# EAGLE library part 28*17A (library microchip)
CMOS EEPROM 16 K (2 K x 8)
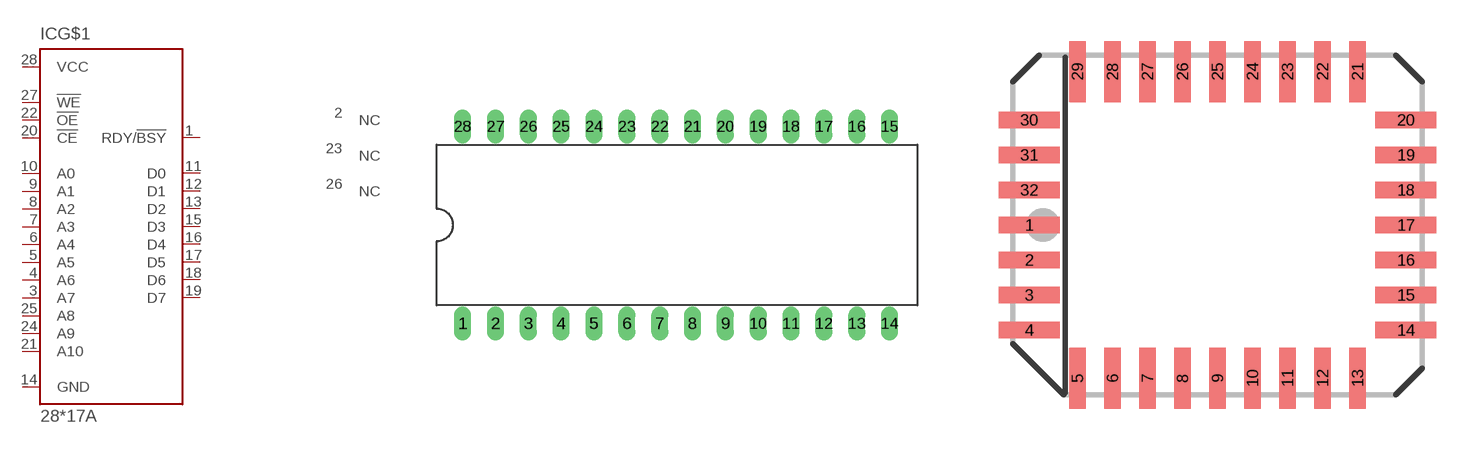
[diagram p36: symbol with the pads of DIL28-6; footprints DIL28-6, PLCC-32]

Designator prefix IC; gates G$1=28C17 2=NC 23=NC 26=NC

## 28C17AP (MPN: CAT28C17ALI20; OC_FARNELL: unknown; OC_NEWARK: 71R7405)  [DIL28-6]
1  G$1:RDY/!BSY  out
2  2:NC  nc
3  G$1:A7  in
4  G$1:A6  in
5  G$1:A5  in
6  G$1:A4  in
7  G$1:A3  in
8  G$1:A2  in
9  G$1:A1  in
10  G$1:A0  in
11  G$1:D0  hiz
12  G$1:D1  hiz
13  G$1:D2  hiz
14  G$1:GND  pwr
15  G$1:D3  hiz
16  G$1:D4  hiz
17  G$1:D5  hiz
18  G$1:D6  hiz
19  G$1:D7  hiz
20  G$1:!CE  in
21  G$1:A10  in
22  G$1:!OE  in
23  23:NC  nc
24  G$1:A9  in
25  G$1:A8  in
26  26:NC  nc
27  G$1:!WE  in
28  G$1:VCC  pwr

## 28C17AL (OC_FARNELL: unknown; OC_NEWARK: unknown)  [PLCC-32]
1  2:NC  nc
2  G$1:RDY/!BSY  out
3  23:NC  nc
4  G$1:A7  in
5  G$1:A6  in
6  G$1:A5  in
7  G$1:A4  in
8  G$1:A3  in
9  G$1:A2  in
10  G$1:A1  in
11  G$1:A0  in
12  26:NC  nc
13  G$1:D0  hiz
14  G$1:D1  hiz
15  G$1:D2  hiz
16  G$1:GND  pwr
18  G$1:D3  hiz
19  G$1:D4  hiz
20  G$1:D5  hiz
21  G$1:D6  hiz
22  G$1:D7  hiz
23  G$1:!CE  in
24  G$1:A10  in
25  G$1:!OE  in
28  G$1:A9  in
29  G$1:A8  in
31  G$1:!WE  in
32  G$1:VCC  pwr

## 28C17AVS (OC_FARNELL: unknown; OC_NEWARK: unknown)  [VSOP28-8X13]
Pads as for DIL28-6

## 28C17ATS (OC_FARNELL: unknown; OC_NEWARK: unknown)  [TSOP28]
1  G$1:!OE  in
2  2:NC  nc
3  G$1:A9  in
4  G$1:A8  in
5  23:NC  nc
6  G$1:!WE  in
7  G$1:VCC  pwr
8  G$1:RDY/!BSY  out
9  26:NC  nc
10  G$1:A7  in
11  G$1:A6  in
12  G$1:A5  in
13  G$1:A4  in
14  G$1:A3  in
15  G$1:A2  in
16  G$1:A1  in
17  G$1:A0  in
18  G$1:D0  hiz
19  G$1:D1  hiz
20  G$1:D2  hiz
21  G$1:GND  pwr
22  G$1:D3  hiz
23  G$1:D4  hiz
24  G$1:D5  hiz
25  G$1:D6  hiz
26  G$1:D7  hiz
27  G$1:!CE  in
28  G$1:A10  in

## 28C17ASO (OC_FARNELL: unknown; OC_NEWARK: unknown)  [SO28W]
Pads as for DIL28-6

## Footprint DIL28-6 (pad centres in mm)
Dual In Line package type P
drill 0.813 long: 1 -16.51,-7.62; 2 -13.97,-7.62; 3 -11.43,-7.62; 4 -8.89,-7.62; 5 -6.35,-7.62; 6 -3.81,-7.62; 7 -1.27,-7.62; 8 1.27,-7.62; 9 3.81,-7.62; 10 6.35,-7.62; 11 8.89,-7.62; 12 11.43,-7.62; 13 13.97,-7.62; 14 16.51,-7.62; 15 16.51,7.62; 16 13.97,7.62; 17 11.43,7.62; 18 8.89,7.62; 19 6.35,7.62; 20 3.81,7.62; 21 1.27,7.62; 22 -1.27,7.62; 23 -3.81,7.62; 24 -6.35,7.62; 25 -8.89,7.62; 26 -11.43,7.62; 27 -13.97,7.62; 28 -16.51,7.62

## Footprint PLCC-32 (pad centres in mm)
PLASTIC LEADED CHIP CARRIER rectangle, package type L
smd 2.2 x 0.6: 1 -6.83,0; 2 -6.83,-1.27; 3 -6.83,-2.54; 4 -6.83,-3.81; 14 6.83,-3.81; 15 6.83,-2.54; 16 6.83,-1.27; 17 6.83,0; 18 6.83,1.27; 19 6.83,2.54; 20 6.83,3.81; 30 -6.83,3.81; 31 -6.83,2.54; 32 -6.83,1.27
smd 0.6 x 2.2: 5 -5.08,-5.56; 6 -3.81,-5.56; 7 -2.54,-5.56; 8 -1.27,-5.56; 9 0,-5.56; 10 1.27,-5.56; 11 2.54,-5.56; 12 3.81,-5.56; 13 5.08,-5.56; 21 5.08,5.56; 22 3.81,5.56; 23 2.54,5.56; 24 1.27,5.56; 25 0,5.56; 26 -1.27,5.56; 27 -2.54,5.56; 28 -3.81,5.56; 29 -5.08,5.56

## Footprint VSOP28-8X13 (pad centres in mm)
Very Small Outline Package 8 x 13.4 mm, package type VS
smd 0.3 x 1.1: 1 0.275,-6.45; 2 0.825,-6.45; 3 1.375,-6.45; 4 1.925,-6.45; 5 2.475,-6.45; 6 3.025,-6.45; 7 3.575,-6.45; 8 3.575,6.45; 9 3.025,6.45; 10 2.475,6.45; 11 1.925,6.45; 12 1.375,6.45; 13 0.825,6.45; 14 0.275,6.45; 15 -0.275,6.45; 16 -0.825,6.45; 17 -1.375,6.45; 18 -1.925,6.45; 19 -2.475,6.45; 20 -3.025,6.45; 21 -3.575,6.45; 22 -3.575,-6.45; 23 -3.025,-6.45; 24 -2.475,-6.45; 25 -1.925,-6.45; 26 -1.375,-6.45; 27 -0.825,-6.45; 28 -0.275,-6.45

## Footprint TSOP28 (pad centres in mm)
Thin Small Outline Package Gull Wing type I, package type TS
smd 0.3 x 1: 1 -3.75,-9.7; 2 -3.25,-9.7; 3 -2.75,-9.7; 4 -2.25,-9.7; 5 -1.75,-9.7; 6 -1.25,-9.7; 7 -0.75,-9.7; 8 0.75,-9.7; 9 1.25,-9.7; 10 1.75,-9.7; 11 2.25,-9.7; 12 2.75,-9.7; 13 3.25,-9.7; 14 3.75,-9.7; 15 3.75,9.7; 16 3.25,9.7; 17 2.75,9.7; 18 2.25,9.7; 19 1.75,9.7; 20 1.25,9.7; 21 0.75,9.7; 22 -0.75,9.7; 23 -1.25,9.7; 24 -1.75,9.7; 25 -2.25,9.7; 26 -2.75,9.7; 27 -3.25,9.7; 28 -3.75,9.7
